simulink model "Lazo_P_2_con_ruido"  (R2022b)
settings: Solver=ode4  StartTime=0.0  StopTime=0.2  FixedStep=1e-6  RelTol=1e-3
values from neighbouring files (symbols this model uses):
  Delta_v_d_2 = P_Delta_v_d_2*v_d_2    [IP_Lazo_P_2.m]    (also in IP_Lazo_Q_12.m = P_Delta_v_d_2*v_d_12)
  I_Delta_v_d_2 = 0.15    [IP_Lazo_P_2.m]    (also in IP_Lazo_Q_12.m)
  Ki_P = ((2+3*v_d_2*Kp_P)/(3*v_d_2*tau))    [IP_Lazo_P_2.m]    (also in Sistema_control_no_lineal_LQR.m = ((2+3*v_d_2*Kp_P)/(3*v_d_2*tau_P)); Sistema_control_no_lineal_Modal.m = ((2+3*v_d_2*Kp_P)/(3*v_d_2*tau_P)))
  Kp_P = 1    [IP_Lazo_P_2.m]    (also in Sistema_control_no_lineal_LQR.m = 0.0002; Sistema_control_no_lineal_Modal.m = 0.0002)
  lim_i_d_2_lower = -75.07117    [IP_Lazo_P_2.m]    (also in Sistema_control_no_lineal_LQR.m; Sistema_control_no_lineal_Modal.m)
  lim_i_d_2_upper = 75.07117    [IP_Lazo_P_2.m]    (also in Sistema_control_no_lineal_LQR.m; Sistema_control_no_lineal_Modal.m)
  P_2_1 = -3000    [IP_Lazo_P_2.m]    (also in Sistema_control_no_lineal_LQR.m; Sistema_control_no_lineal_Modal.m)
  P_2_2 = 3000    [IP_Lazo_P_2.m]    (also in Sistema_control_no_lineal_LQR.m; Sistema_control_no_lineal_Modal.m)
  v_d_2 = 100*sqrt(2)    [IP_Lazo_P_2.m]    (also in Sistema_no_lineal_Modal.m; Sistema_no_lineal_LQR.m; Sistema_control_no_lineal_LQR.m; Sistema_control_no_lineal_Modal.m)
  V_R_P = D_R_P^2    (= 0.0009)    [IP_Lazo_P_2.m]

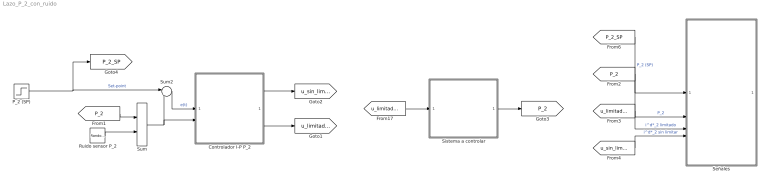
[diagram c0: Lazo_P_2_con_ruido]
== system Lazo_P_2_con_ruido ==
  Controlador I-P P_2 : Subsystem
  P_2 (SP) : Step  Time=0.1  Before=P_2_1  After=P_2_2  SampleTime=0
  Ruido sensor P_2 : RandomNumber  Variance=V_R_P  SampleTime=0.00011
  Señales : Subsystem
  Sistema a controlar : Subsystem
  Sum : Sum
  Sum2 : Sum  Inputs=|+-
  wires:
  P_2 (SP)/1 -> [P_2_SP], Sum2/1  "Set-point"
  Sum2/1 -> Controlador I-P P_2/1(e(t))  "e(t)"
  Controlador I-P P_2/2(i^d*_2 limitado) -> [u_limitado_2]
  Controlador I-P P_2/1(i^d*_2 sin limitar) -> [u_sin_limitar_2]
  [u_limitado_2] -> Sistema a controlar/1(i^d*_2 limitado)
  Sistema a controlar/1(P_2) -> [P_2]
  [P_2_SP] -> Señales/1(P_2 (SP))  "P_2 (SP)"
  [P_2] -> Señales/2(P_2)  "P_2"
  [u_limitado_2] -> Señales/3(i^d*_2 limitado)  "i^d*_2 limitado"
  [u_sin_limitar_2] -> Señales/4(i^d*_2 sin limitar)  "i^d*_2 sin limitar"
  Sum/1 -> Sum2/2, Controlador I-P P_2/2(P_2)
  Ruido sensor P_2/1 -> Sum/2
  [P_2] -> Sum/1

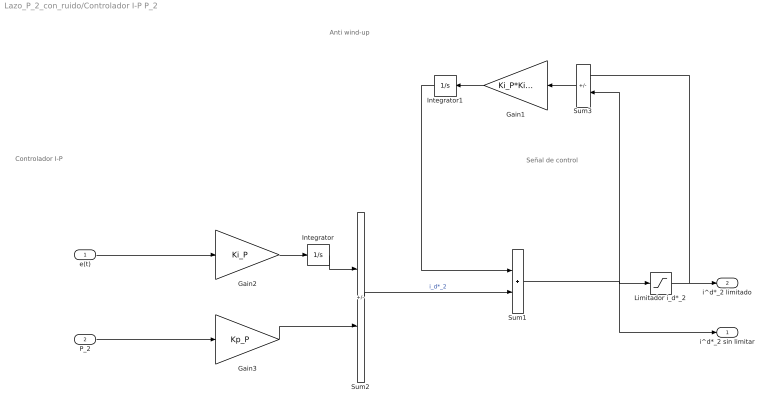
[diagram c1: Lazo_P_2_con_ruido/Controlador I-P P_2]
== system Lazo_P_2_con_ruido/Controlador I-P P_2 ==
  note: Señal de control
  note: Controlador I-P
  note: Anti wind-up
  e(t) : Inport
  P_2 : Inport  Port=2
  Gain1 : Gain  Gain=Ki_P*Ki_P
  Gain2 : Gain  Gain=Ki_P
  Gain3 : Gain  Gain=Kp_P
  Integrator : Integrator
  Integrator1 : Integrator
  Limitador i_d*_2 : Saturate  UpperLimit=lim_i_d_2_upper  LowerLimit=lim_i_d_2_lower
  Sum1 : Sum
  Sum2 : Sum  Inputs=+-
  Sum3 : Sum  Inputs=+-
  i^d*_2 sin limitar : Outport
  i^d*_2 limitado : Outport  Port=2
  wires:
  Limitador i_d*_2/1 -> i^d*_2 limitado/1, Sum3/1
  Sum1/1 -> i^d*_2 sin limitar/1, Limitador i_d*_2/1, Sum3/2
  Sum2/1 -> Sum1/2  "i_d*_2"
  Gain2/1 -> Integrator/1
  Integrator/1 -> Sum2/1
  e(t)/1 -> Gain2/1
  Sum3/1 -> Gain1/1
  Gain1/1 -> Integrator1/1
  Integrator1/1 -> Sum1/1
  P_2/1 -> Gain3/1
  Gain3/1 -> Sum2/2

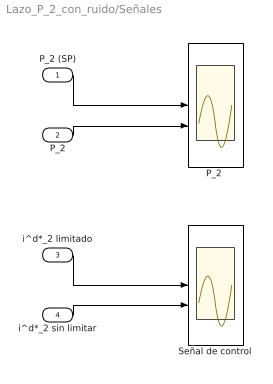
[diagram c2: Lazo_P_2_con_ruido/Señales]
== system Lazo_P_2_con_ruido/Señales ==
  P_2 (SP) : Inport
  P_2 : Inport  Port=2
  i^d*_2 limitado : Inport  Port=3
  i^d*_2 sin limitar : Inport  Port=4
  "P_2 " : Scope  NumInputPorts=2
  Señal de control : Scope  NumInputPorts=2
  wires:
  P_2 (SP)/1 -> "P_2 "/1
  i^d*_2 sin limitar/1 -> Señal de control/2
  i^d*_2 limitado/1 -> Señal de control/1
  P_2/1 -> "P_2 "/2

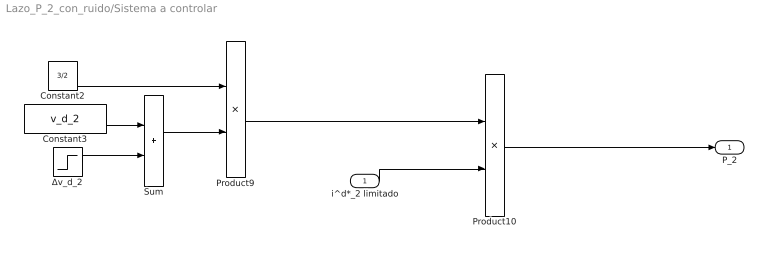
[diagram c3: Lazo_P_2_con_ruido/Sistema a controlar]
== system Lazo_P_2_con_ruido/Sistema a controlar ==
  i^d*_2 limitado : Inport
  Constant2 : Constant  Value=3/2
  Constant3 : Constant  Value=v_d_2
  Product10 : Product
  Product9 : Product
  Sum : Sum
  Δv_d_2 : Step  Time=I_Delta_v_d_2  After=Delta_v_d_2  SampleTime=0
  P_2 : Outport
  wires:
  Product9/1 -> Product10/1
  i^d*_2 limitado/1 -> Product10/2
  Product10/1 -> P_2/1
  Δv_d_2/1 -> Sum/2
  Constant2/1 -> Product9/1
  Sum/1 -> Product9/2
  Constant3/1 -> Sum/1
